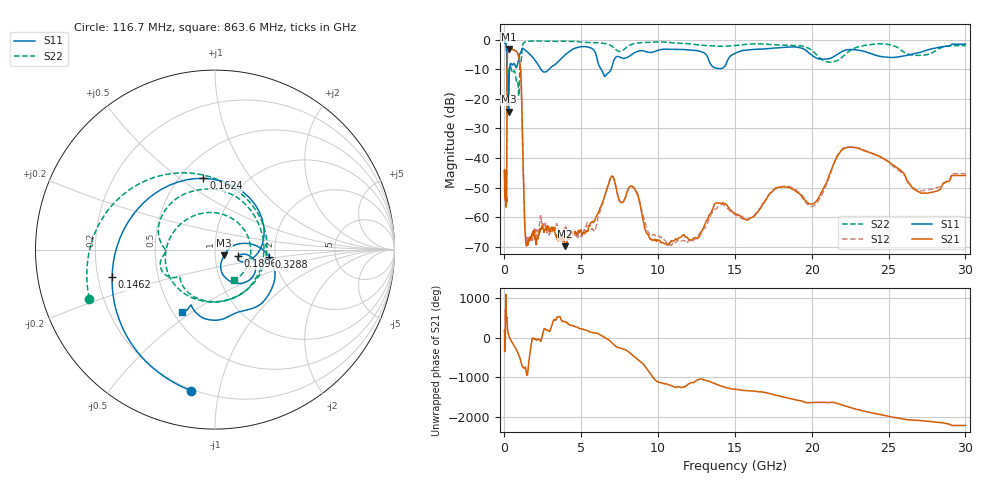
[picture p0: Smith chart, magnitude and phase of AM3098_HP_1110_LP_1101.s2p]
! Date/Time: Thu, Feb 28, 2019 8:47 AM
! Network Analyzer: Agilent Technologies E8364B Rev: A.07.50.67
! Sweep from 0.010 to 30.000 GHz, 1601 Points, Sweep Type: LOG
! Power Supply: 5.022 V, 0.002 A
# Hz S DB R 50
!freq MagS11 AngS11 MagS21 AngS21 MagS12 AngS12 MagS22 AngS22
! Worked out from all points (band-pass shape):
!   1601 points, 10 MHz to 30 GHz, reference 50 ohm
!   highest |S21| = -3.13 dB at 293 MHz (marker M1); lowest = -69.8 dB at 3.953 GHz (marker M2)
!   |S21| within 3 dB of the highest: 183.7 MHz to 945.1 MHz (761.3 MHz wide, 135 % of centre)
!   lowest |S11| = -24.4 dB at 265.1 MHz (marker M3), VSWR 1.13, Z = 55.3 - j3.46 ohm
!   |S11| at or under -10 dB: 169.7 MHz to 333.1 MHz (163.4 MHz wide, 65 % of centre); 2.372 GHz to 2.899 GHz (527 MHz wide, 20 % of centre); 6.289 GHz to 6.94 GHz (650.8 MHz wide, 9.84 % of centre)
!   |S22| runs from -19.1 to -0.4 dB; largest |S21 - S12| = 0.012
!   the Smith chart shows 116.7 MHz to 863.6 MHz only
!   S11 on the Smith chart (normalised r, x): 116.7 MHz: 0.19, -0.83; 146.2 MHz: 0.26, -0.12; 162.4 MHz: 0.65, +0.62; 189.6 MHz: 1.29, -0.10; 328.8 MHz: 1.86, -0.16; 863.6 MHz: 0.56, -0.46
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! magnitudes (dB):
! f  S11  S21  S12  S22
! 10 MHz  -0.4  -44.2  -45.2  -0.6
! 38.04 MHz  -0.3  -50.4  -51.5  -0.8
! 116.7 MHz  -2.0  -54.3  -54.7  -2.5
! 144.7 MHz  -4.3  -50.8  -50.5  -5.4
! 146.2 MHz  -4.5  -49.5  -49.4  -5.8
! 162.4 MHz  -7.9  -22.3  -22.2  -10.8
! 189.6 MHz  -17.4  -5.2  -5.2  -12.0
! 265.1 MHz  -24.4  -3.2  -3.2  -11.2
! 293 MHz  -15.8  -3.1  -3.1  -10.8
! 328.8 MHz  -10.3  -3.2  -3.2  -9.5
! 550.5 MHz  -8.4  -3.4  -3.4  -11.0
! 863.6 MHz  -8.1  -4.7  -4.7  -13.9
! 1.076 GHz  -4.2  -12.6  -12.6  -7.5
! 1.382 GHz  -3.7  -68.4  -67.0  -0.7
! 2.084 GHz  -7.6  -69.3  -64.9  -0.4
! 3.953 GHz  -5.1  -69.8  -63.6  -0.6
! 7.926 GHz  -6.1  -52.4  -52.5  -2.7
! 11.03 GHz  -3.3  -68.1  -69.2  -1.1
! 20.1 GHz  -5.6  -55.6  -56.3  -4.0
! 22.56 GHz  -3.3  -36.4  -36.2  -3.5
! 27.28 GHz  -3.9  -51.9  -51.1  -5.3
! 30 GHz  -1.6  -45.9  -45.3  -2.1
